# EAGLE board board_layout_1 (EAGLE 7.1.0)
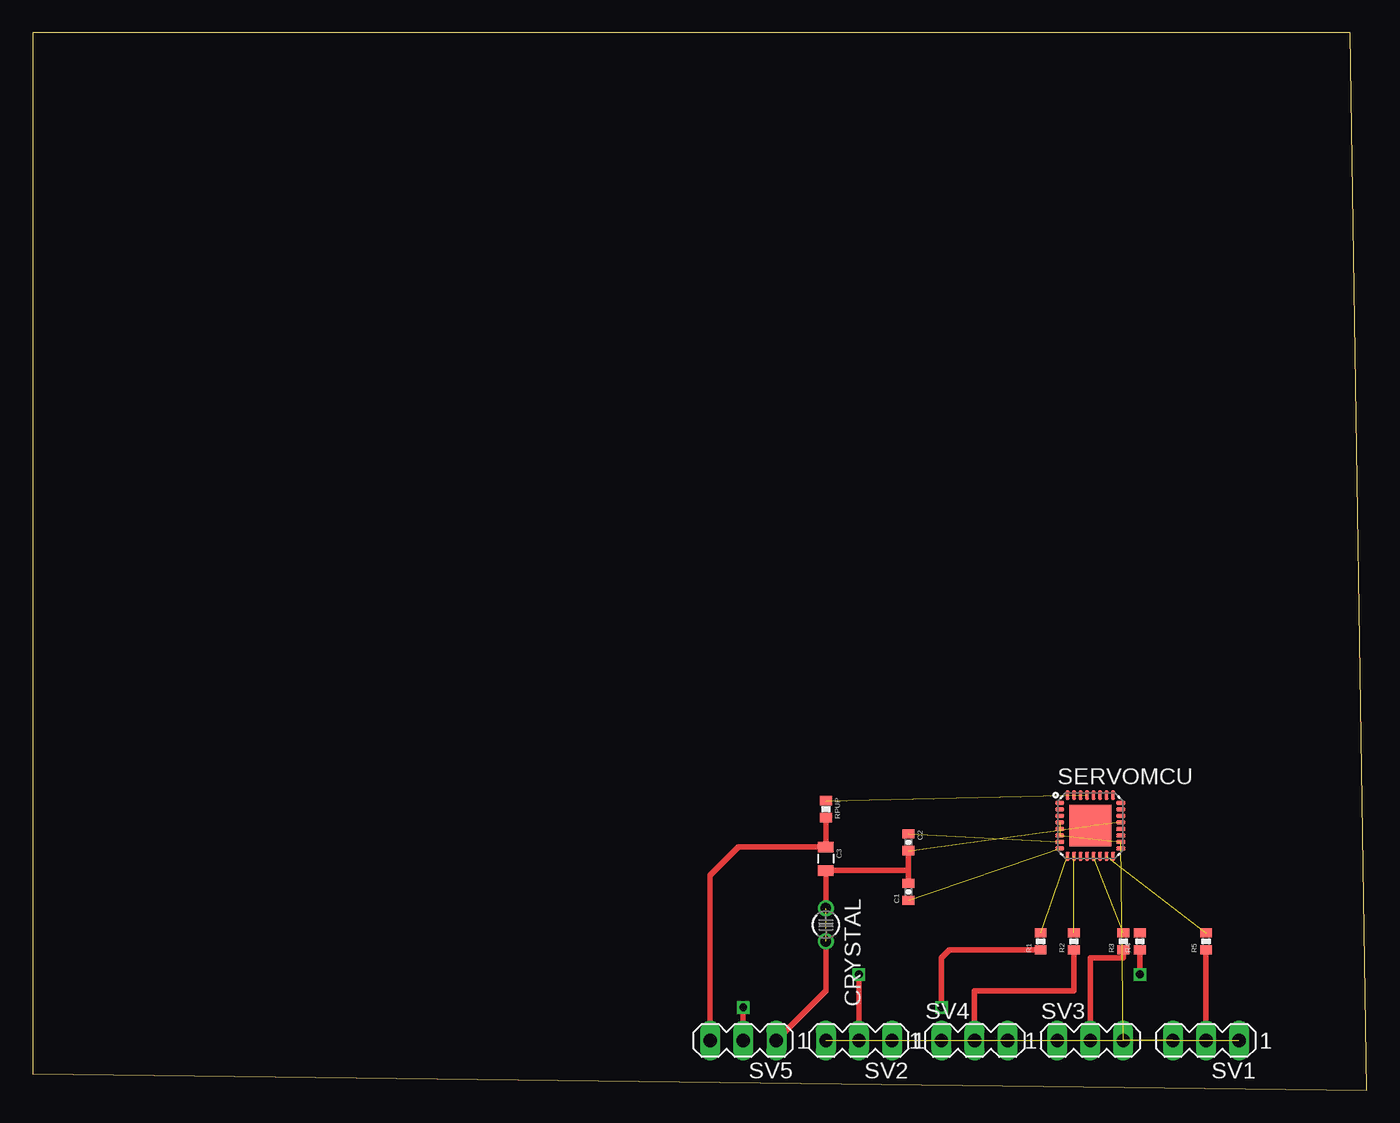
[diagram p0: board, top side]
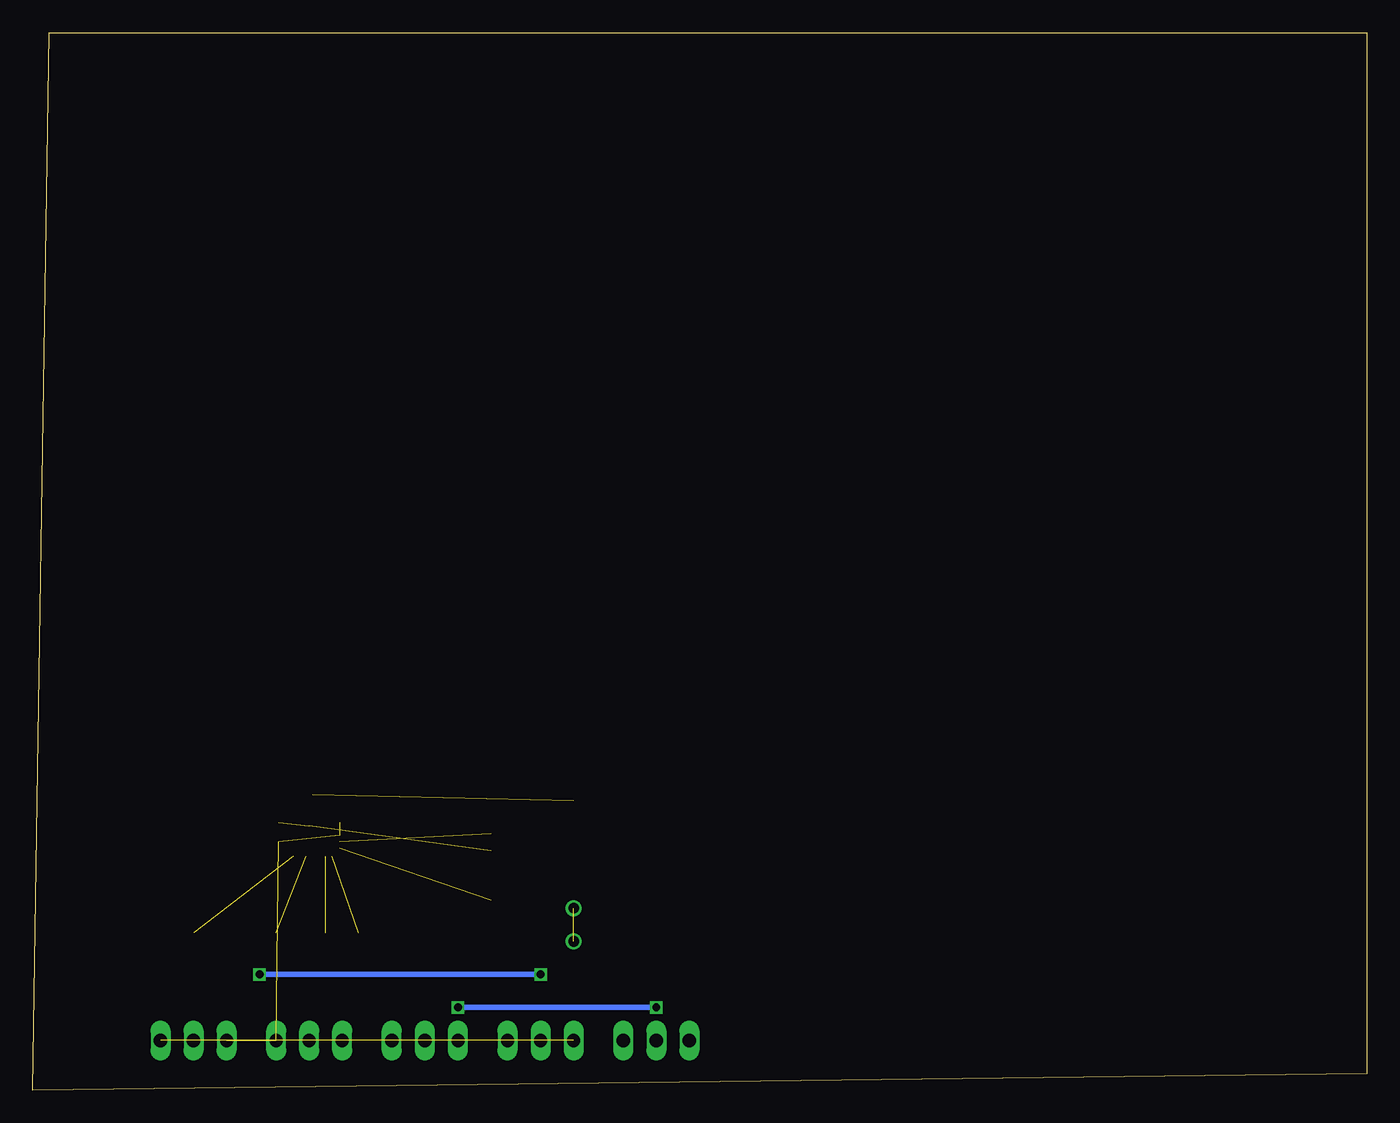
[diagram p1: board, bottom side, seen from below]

Size 102.54 x 81.27 mm. Coordinates in mm from the lower left corner, seen from the top.
Outline: 0,1.27 102.54,0 101.27,81.27 0,81.27 0,1.27
Copper layers (1*16): Top 0.0356mm / dielectric 1.5011mm / Bottom 0.0356mm
Design rules "LaenPCBOrder": minimum track width 6mil, minimum drill 13mil, track to track 6mil, track to pad 6mil, pad to pad 6mil, via to via 6mil, smd to smd 6mil, copper to edge 15mil, drill to drill 6mil, minimum pad ring 7mil, minimum via ring 7mil, stop-mask expansion 3mil, vias tented up to drill 0mil, thermal gap 10mil

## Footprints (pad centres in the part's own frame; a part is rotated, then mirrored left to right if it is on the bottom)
0402-CAP = smd 0.7 x 0.9: 1 -0.65,0; 2 0.65,0
0805 = smd 0.8 x 1.2: 1 -0.9,0; 2 0.9,0
TC26V = drill 0.813: 1 -1.27,0; 2 1.27,0
0402-RES = smd 0.7 x 0.9: 1 -0.65,0; 2 0.65,0
MLF32-PAD = smd 0.7 x 0.3: 1 -2.35,1.75; 2 -2.35,1.25; 3 -2.35,0.75; 4 -2.35,0.25; 5 -2.35,-0.25; 6 -2.35,-0.75; 7 -2.35,-1.25; 8 -2.35,-1.75; 17 2.35,-1.75; 18 2.35,-1.25; 19 2.35,-0.75; 20 2.35,-0.25; 21 2.35,0.25; 22 2.35,0.75; 23 2.35,1.25; 24 2.35,1.75 | smd 0.3 x 0.7: 9 -1.75,-2.35; 10 -1.25,-2.35; 11 -0.75,-2.35; 12 -0.25,-2.35; 13 0.25,-2.35; 14 0.75,-2.35; 15 1.25,-2.35; 16 1.75,-2.35; 25 1.75,2.35; 26 1.25,2.35; 27 0.75,2.35; 28 0.25,2.35; 29 -0.25,2.35; 30 -0.75,2.35; 31 -1.25,2.35; 32 -1.75,2.35 | smd 3.2 x 3.2: PAD 0,0
MA03-1 = drill 1.016 long: 1 -2.54,0; 2 0,0; 3 2.54,0

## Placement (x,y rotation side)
C1  22pf  [0402-CAP]  67.31,15.24 90 top
C2  22pf  [0402-CAP]  67.31,19.05 270 top
C3  [0805]  60.96,17.78 270 top
CRYSTAL  16MHz  [TC26V]  60.96,12.7 270 top
R1  1k  [0402-RES]  77.47,11.43 90 top
R2  1k  [0402-RES]  80.01,11.43 90 top
R3  1k  [0402-RES]  83.82,11.43 90 top
R4  1k  [0402-RES]  85.09,11.43 90 top
R5  1k  [0402-RES]  90.17,11.43 90 top
RPUP  10k  [0402-RES]  60.96,21.59 270 top
SERVOMCU  atmega328p  [MLF32-PAD]  81.28,20.32 0 top
SV1  sv1  [MA03-1]  90.17,3.81 180 top
SV2  sv2  [MA03-1]  63.5,3.81 180 top
SV3  sv3  [MA03-1]  81.28,3.81 0 top
SV4  sv4  [MA03-1]  72.39,3.81 0 top
SV5  sv5  [MA03-1]  54.61,3.81 180 top

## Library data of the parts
C1 C2 R1-R5 RPUP = SparkFun-Passives
C3 = SparkFun-Capacitors
CRYSTAL = crystal; OC_FARNELL: unknown; OC_NEWARK: unknown
SERVOMCU = SparkFun-DigitalIC
SV1-SV5 = con-lstb; OC_FARNELL: unknown; OC_NEWARK: unknown

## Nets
GND: C1.2 C2.2 C3.2 CRYSTAL.1 CRYSTAL.2 SERVOMCU.21 SERVOMCU.PAD SV5.1
N$1: R5.2 SERVOMCU.15
N$2: SERVOMCU.14
N$3: R3.2 SERVOMCU.13
N$4: RPUP.1 SERVOMCU.29
N$5: R2.1 SV4.2
N$6: R1.1 SV5.2
N$7: R2.2 SERVOMCU.10
N$8: R1.2 SERVOMCU.9
N$9: R3.1 SV3.2
N$10: C1.1 SERVOMCU.8
N$11: C2.1 SERVOMCU.7
N$12: R5.1 SV1.2
N$13: R4.1 SV2.2
N$14: SERVOMCU.4 SERVOMCU.6 SERVOMCU.18 SV1.3 SV3.3
N$15: SV2.3 SV4.3
N$16: SV1.1 SV2.1 SV3.1 SV4.1
N$17: SERVOMCU.5
VCC: C3.1 RPUP.2 SV5.3

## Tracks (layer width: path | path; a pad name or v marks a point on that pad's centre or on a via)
GND  (3 unrouted)
  Top 0.406: CRYSTAL.1 C3.2 67.31,16.88 | C1.2 67.31,16.88 | 67.31,16.88 C2.2 | SV5.1 60.96,7.62 CRYSTAL.2
N$1  (1 unrouted)
N$3  (1 unrouted)
N$4  (1 unrouted)
N$5
  Top 0.406: R2.1 80.01,7.62 72.39,7.62 SV4.2
N$6  (via drill 0.6)
  Top 0.406: SV5.2 v54.61,6.35 | v69.85,6.35 69.85,10.16 70.47,10.78 R1.1
  Bottom 0.406: v54.61,6.35 v69.85,6.35
N$7  (1 unrouted)
N$8  (1 unrouted)
N$9
  Top 0.406: SV3.2 81.28,10.16 83.82,10.16 R3.1
N$10  (1 unrouted)
N$11  (1 unrouted)
N$12
  Top 0.406: R5.1 SV1.2
N$13  (via drill 0.6)
  Top 0.406: R4.1 v85.09,8.89 | v63.5,8.89 SV2.2
  Bottom 0.406: v85.09,8.89 v63.5,8.89
N$14  (4 unrouted)
N$15  (1 unrouted)
N$16  (3 unrouted)
VCC
  Top 0.406: RPUP.2 C3.1 54.24,18.68 52.07,16.51 SV5.3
